(* Logix 5000 AddOnInstructionDefinition export AMCI_MSO_Enable; software revision 20.05 *)

TYPE AMCI_Motion_Axis_Output_Data :
STRUCT
   Control_Word_0 : INT;
   Control_Word_1 : INT;
   Position_or_Distance : DINT;
   Programmed_Speed : DINT;
   Acceleration : INT;
   Deceleration : INT;
   Output_Word_8 : INT;
   Output_Word_9 : INT;
END_STRUCT
END_TYPE

TYPE AMCI_Motion_Axis_Input_Data :
STRUCT
   Moving_CW : BOOL;
   Moving_CCW : BOOL;
   In_Hold_State : BOOL;
   Stopped : BOOL;
   At_Home : BOOL;
   Accelerating : BOOL;
   Decelerating : BOOL;
   Move_Complete : BOOL;
   Status_Word_0_Bit_8 : BOOL;
   Status_Word_0_Bit_9 : BOOL;
   Position_Invalid : BOOL;
   Input_Error : BOOL;
   Command_Error : BOOL;
   Configuration_Error : BOOL;
   Module_OK : BOOL;
   Mode_Flag : BOOL;
   IN1_Active : BOOL;
   IN2_Active : BOOL;
   IN3_Active : BOOL;
   IN4_Active : BOOL;
   Status_Word_1_Bit_4 : BOOL;
   Status_Word_1_Bit_5 : BOOL;
   Connection_Was_Lost : BOOL;
   Driver_Fault : BOOL;
   Status_Word_1_Bit_8 : BOOL;
   Invalid_Jog_Change : BOOL;
   Status_Word_1_Bit_10 : BOOL;
   Heartbeat_Bit : BOOL;
   Status_Word_1_Bit_12 : BOOL;
   Status_Word_1_Bit_13 : BOOL;
   Stall_Detected : BOOL;
   Drive_Is_Enabled : BOOL;
   Motor_Position : DINT;
   Encoder_Position : DINT;
   Trapped_Encoder_Position : DINT;
   Input_Word_8 : INT;
   Input_Word_9 : INT;
END_STRUCT
END_TYPE

ADD_ON_INSTRUCTION AMCI_MSO_Enable   (* revision 1.0, vendor AMCI, ExecuteEnableInFalse *)
// AMCI Enable Driver
// Help:
// MSO_ENABLE:   Sends power to the motor.
// This instruction must only be used to change the existing enabled / disabled state of the AMCI motion device.  It MUST NOT be used in an unconditional rung because it will interfere with the other instructions sending data to the motion device
// AXIS INPUT DATA:  Input data from AMCI motion device.   Uses the AMCI_Motion_Axis_Input_Data User Defined Data Type.
// AXIS OUTPUT DATA; Output data from the AOI to the AMCI motion device.   Uses the AMCI_Motion_Axis_Output_Data User Defined Data Type.
// EN (Enable) Set when rung is true, Reset when rung is false
// DN (Done) Set when command is sent to the motion device.  Reset when the rung is false.
VAR_IN_OUT
   Axis_Input_Data : AMCI_Motion_Axis_Input_Data; {required}
        [0].6   // set when decelerating
   Axis_Output_Data : AMCI_Motion_Axis_Output_Data; {required}
END_VAR
VAR_OUTPUT
   EN : BOOL; {visible}   // set when rung with AOI is true
   DN : BOOL; {access Read Only, visible}   // set when reset error command sent to motion axis
END_VAR
VAR
   command_data_block : INT[10];
        [0]   // Command Bits MSW
        [1]   // Command Bits LSW
        [2]   // Upper Target Position
        [3]   // Lower Target Position
        [4]   // Upper Programmed Speed
        [5]   // Lower Programmed Speed
END_VAR

ROUTINE EnableInFalse   (* ladder *)
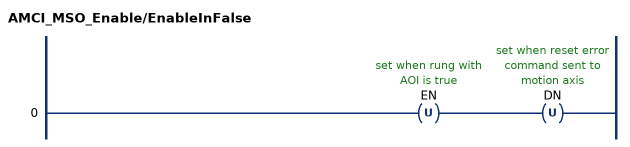
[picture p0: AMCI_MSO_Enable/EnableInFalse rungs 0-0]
   0: OTU(EN)OTU(DN);
END_ROUTINE

ROUTINE Logic   (* ladder *)
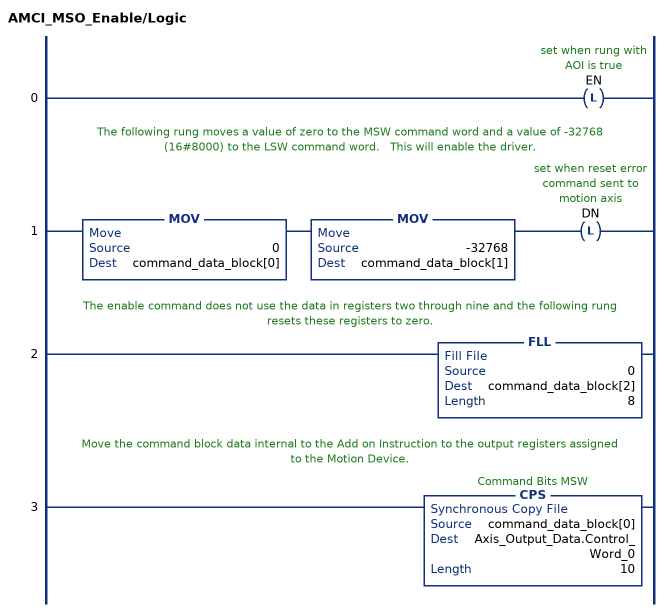
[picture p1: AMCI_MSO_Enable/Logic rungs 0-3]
   0: OTL(EN);
   // The following rung moves a value of zero to the MSW command word and a value of -32768 (16#8000) to the LSW command word.   This will enable the driver.
   1: MOV(0,command_data_block[0])MOV(-32768,command_data_block[1])OTL(DN);
   // The enable command does not use the data in registers two through nine and the following rung resets these registers to zero.
   2: FLL(0,command_data_block[2],8);
   // Move the command block data internal to the Add on Instruction to the output registers assigned to the Motion Device.
   3: CPS(command_data_block[0],Axis_Output_Data.Control_Word_0,10);
END_ROUTINE
END_ADD_ON_INSTRUCTION
